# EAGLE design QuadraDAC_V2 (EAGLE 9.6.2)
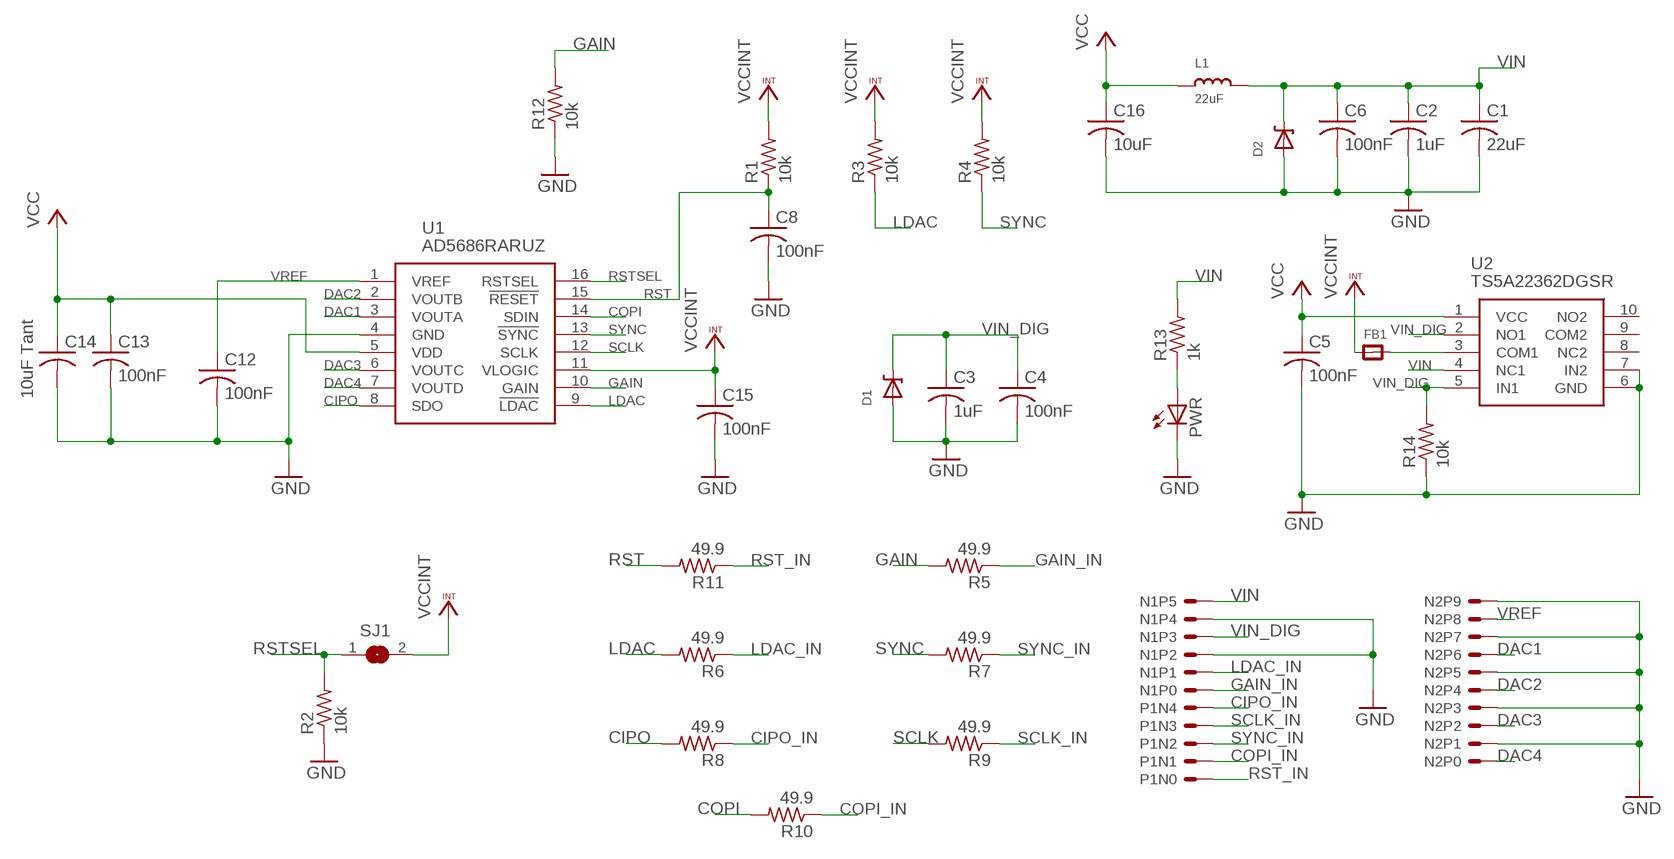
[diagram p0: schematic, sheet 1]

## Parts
C1  22uF  C-USC0603  [C0603]
C2  1uF  C-USC0603  [C0603]
C3  1uF  C-USC0603  [C0603]
C4  100nF  C-USC0603  [C0603]
C5  100nF  C-USC0603  [C0603]
C6  100nF  C-USC0603  [C0603]
C8  100nF  C-USC0603  [C0603]
C12  100nF  C-USC0603  [C0603]
C13  100nF  C-USC0603  [C0603]
C14  10uF Tant  C-USC0805  [C0805]
C15  100nF  C-USC0603  [C0603]
C16  10uF  C-USC0603  [C0603]
D1  DDZ5V6ASF  [DDZ5V6ASF]
D2  DDZ5V6ASF  [DDZ5V6ASF]
FB1  FERRITE_0603  [_0603]
L1  22uF  INDUCTOR0805  [0805]
N1  6PINHEADER  [6PINHEADER]
N2  10PINHEADER  [10PINHEADER]
P1  5PINHEADER  [5PINHEADER]
PWR  LEDCHIPLED_0603  [CHIPLED_0603]
R1  10k  R-US_R0603  [R0603]
R2  10k  R-US_R0603  [R0603]
R3  10k  R-US_R0603  [R0603]
R4  10k  R-US_R0603  [R0603]
R5  49.9  R-US_R0603  [R0603]
R6  49.9  R-US_R0603  [R0603]
R7  49.9  R-US_R0603  [R0603]
R8  49.9  R-US_R0603  [R0603]
R9  49.9  R-US_R0603  [R0603]
R10  49.9  R-US_R0603  [R0603]
R11  49.9  R-US_R0603  [R0603]
R12  10k  R-US_R0603  [R0603]
R13  1k  R-US_R0603  [R0603]
R14  10k  R-US_R0603  [R0603]
SJ1  SOLDERJUMPER  [SOLDERJUMPER_ARROW_NOPASTE]
U1  AD5686RARUZ  [SOP65P640X120-16N]
U2  TS5A22362DGSR  [SOP50P490X110-10N]

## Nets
CIPO: R8.2 U1.8(SDO)
CIPO_IN: P1.N4 R8.1
COPI: R10.2 U1.14(SDIN)
COPI_IN: P1.N1 R10.1
DAC1: N2.P6 U1.3(VOUTA)
DAC2: N2.P4 U1.2(VOUTB)
DAC3: N2.P2 U1.6(VOUTC)
DAC4: N2.P0 U1.7(VOUTD)
GAIN: R5.2 R12.2 U1.10(GAIN)
GAIN_IN: N1.P0 R5.1
GND: C1.2 C2.2 C3.2 C4.2 C5.2 C6.2 C8.2 C12.2 C13.2 C14.2 C15.2 C16.2 D1.P$1(A) D2.P$1(A) N1.P2 N1.P4 N2.P1 N2.P3 N2.P5 N2.P7 N2.P9 PWR.C R2.1 R12.1 R14.1 U1.4(GND) U2.6(GND) U2.7(IN2)
LDAC: R3.1 R6.2 U1.9(!LDAC)
LDAC_IN: N1.P1 R6.1
N$1: PWR.A R13.1
N$4: FB1.2 U2.3(COM1)
RST: C8.1 R1.1 R11.2 U1.15(!RESET)
RST_IN: P1.N0 R11.1
RSTSEL: R2.2 SJ1.1 U1.16(RSTSEL)
SCLK: R9.2 U1.12(SCLK)
SCLK_IN: P1.N3 R9.1
SYNC: R4.1 R7.2 U1.13(!SYNC)
SYNC_IN: P1.N2 R7.1
VCC: C5.1 C13.1 C14.1 C16.1 L1.1 U1.5(VDD) U2.1(VCC)
VCCINT: C15.1 FB1.1 R1.2 R3.2 R4.2 SJ1.2 U1.11(VLOGIC)
VIN: C1.1 C2.1 C6.1 D2.P$2(C) L1.2 N1.P5 R13.2 U2.4(NC1)
VIN_DIG: C3.1 C4.1 D1.P$2(C) N1.P3 R14.2 U2.2(NO1) U2.5(IN1)
VREF: C12.1 N2.P8 U1.1(VREF)
Unconnected: U2.8(NC2) U2.9(COM2) U2.10(NO2)

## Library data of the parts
C1-C6 C8 C12-C16 = rcl:C-US: CAPACITOR, American symbol; SPICEPREFIX: C
D1 D2 = ForceTronics:DDZ5V6ASF: DDZ5V6ASF 5.42 Zener Diode
FB1 = microbuilder:FERRITE: Ferrite Bead
L1 = microbuilder:INDUCTOR: Inductors
N1 = ForceTronics-ForceTronics:6PINHEADER
N2 = ForceTronics-ForceTronics:10PINHEADER
P1 = ForceTronics-ForceTronics:5PINHEADER
PWR = adafruit:LED: LED
R1-R14 = rcl:R-US_: RESISTOR, American symbol; SPICEPREFIX: R
SJ1 = microbuilder:SOLDERJUMPER: SMD Solder JUMPER; BOM: EXCLUDE
U1 = SamacSys_Parts:AD5686RARUZ: AD5686RARUZ, 16 bit DAC Quad SPI, 16-pin TSSOP Source: Datasheet; DESCRIPTION: AD5686RARUZ, 16 bit DAC Quad SPI, 16-pin TSSOP; HEIGHT: 1.2mm; MANUFACTURER_NAME: Analog Devices; MANUFACTURER_PART_NUMBER: AD5686RARUZ; MOUSER_PART_NUMBER: 584-AD5686RARUZ; MOUSER_PRICE-STOCK: https://www.mouser.co.uk/ProductDetail/Analog-Devices/AD5686RARUZ?qs=NmRFExCfTkGcAlYhNpYDVg%3D%3D
U2 = SamacSys_Parts:TS5A22362DGSR: Texas Instruments TS5A22362DGSR, Analogue Switch Dual SPDT, 2.3 5.5 V, 10-Pin VSSOP Source: Datasheet; DESCRIPTION: Texas Instruments TS5A22362DGSR, Analogue Switch Dual SPDT, 2.3 5.5 V, 10-Pin VSSOP; HEIGHT: 1.1mm; MANUFACTURER_NAME: Texas Instruments; MANUFACTURER_PART_NUMBER: TS5A22362DGSR; MOUSER_PART_NUMBER: 595-TS5A22362DGSR; MOUSER_PRICE-STOCK: https://www.mouser.co.uk/ProductDetail/Texas-Instruments/TS5A22362DGSR?qs=snW7ThfrdqwrWVQhLBj0GQ%3D%3D

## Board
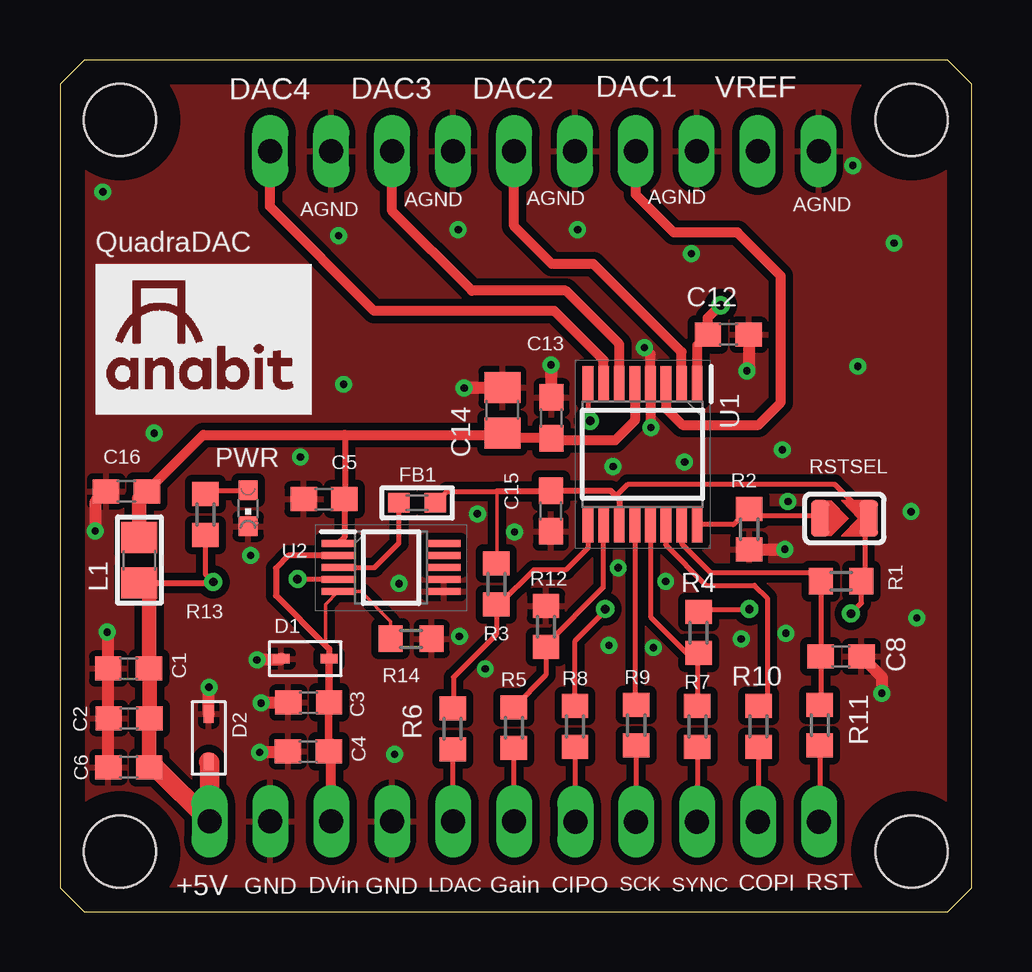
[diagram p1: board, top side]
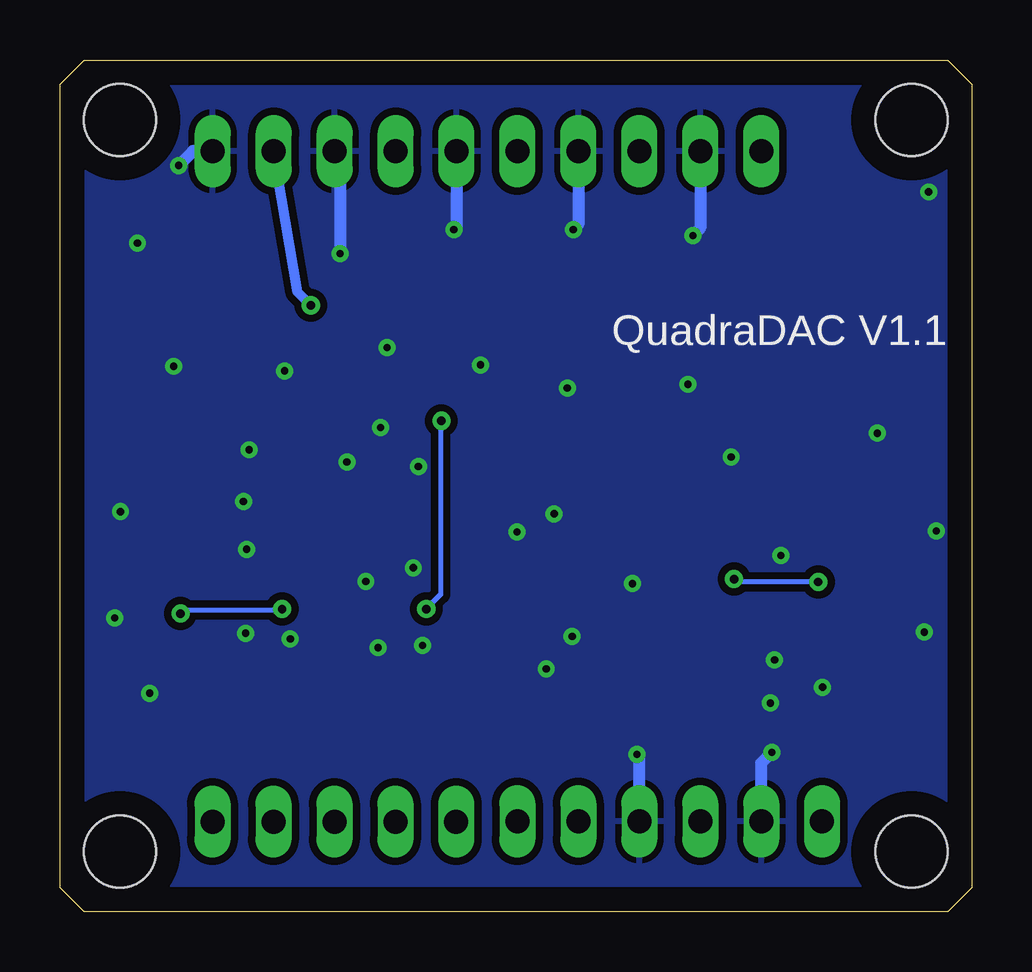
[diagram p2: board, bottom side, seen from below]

Size 38 x 35.5 mm. Coordinates in mm from the lower left corner, seen from the top.
Outline: 38,1 38,34.5 37,35.5 1,35.5 0,34.5 0,1 1,0 37,0 38,1
Copper layers (1*16): Top 0.035mm / dielectric 1.5mm / Bottom 0.035mm
Design rules "default *": minimum track width 6mil, minimum drill 0.3mm, track to track 6mil, track to pad 6mil, pad to pad 6mil, via to via 6mil, smd to smd 6mil, copper to edge 40mil, drill to drill 6mil, minimum pad ring 10mil, minimum via ring 8mil, stop-mask expansion 4mil, vias tented up to drill 0mil, thermal gap 10mil
Holes 3 mm at 2.5,2.5 35.5,2.5 2.5,33 35.5,33

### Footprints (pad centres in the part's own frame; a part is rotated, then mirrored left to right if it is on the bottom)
C0603 = smd 1.1 x 1: 1 -0.85,0; 2 0.85,0
C0805 = smd 1.3 x 1.5: 1 -0.95,0; 2 0.95,0
DDZ5V6ASF = smd 0.71 x 0.41: P$1 0,0; P$2 1.99,0
_0603 = smd 0.9 x 0.8: 1 -0.762,0; 2 0.762,0
0805 = smd 1.3 x 1.5: 1 -0.95,0; 2 0.95,0
6PINHEADER = drill 1 long: P0 1.27,-1.778; P1 3.81,-1.778; P2 6.35,-1.778; P3 8.89,-1.778; P4 11.43,-1.778; P5 13.97,-1.778
10PINHEADER = drill 1 long: P0 1.27,-3.81; P1 3.81,-3.81; P2 6.35,-3.81; P3 8.89,-3.81; P4 11.43,-3.81; P5 13.97,-3.81; P6 16.51,-3.81; P7 19.05,-3.81; P8 21.59,-3.81; P9 24.13,-3.81
5PINHEADER = drill 1 long: N0 -5.08,0; N1 -2.54,0; N2 0,0; N3 2.54,0; N4 5.08,0
CHIPLED_0603 = smd 0.8 x 0.8: A 0,-0.75; C 0,0.75
R0603 = smd 1 x 1.1: 1 -0.85,0; 2 0.85,0
SOLDERJUMPER_ARROW_NOPASTE = smd 0.762 x 1.524: 1 -1.016,0; 2 1.016,0
SOP65P640X120-16N = smd 1.475 x 0.45: 1 -2.938,2.275; 2 -2.938,1.625; 3 -2.938,0.975; 4 -2.938,0.325; 5 -2.938,-0.325; 6 -2.938,-0.975; 7 -2.938,-1.625; 8 -2.938,-2.275; 9 2.938,-2.275; 10 2.938,-1.625; 11 2.938,-0.975; 12 2.938,-0.325; 13 2.938,0.325; 14 2.938,0.975; 15 2.938,1.625; 16 2.938,2.275
SOP50P490X110-10N = smd 1.4 x 0.3: 1 -2.2,1; 2 -2.2,0.5; 3 -2.2,0; 4 -2.2,-0.5; 5 -2.2,-1; 6 2.2,-1; 7 2.2,-0.5; 8 2.2,0; 9 2.2,0.5; 10 2.2,1

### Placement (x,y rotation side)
C1  2.86,10.13 180 top
C2  2.88,8.06 180 top
C3  10.37,8.71 180 top
C4  10.35,6.68 180 top
C5  11.01,17.19 180 top
C6  2.87,6.02 180 top
C8  32.56,10.63 0 top
C12  27.86,24.05 0 top
C13  20.49,20.58 90 top
C14  18.44,20.9 90 top
C15  20.46,16.7 270 top
C16  2.77,17.52 180 top
D1  9.22,10.54 0 top
D2  6.2,8.23 270 top
FB1  14.89,17.04 180 top
L1  3.31,14.65 270 top
N1  20.2,1.98 180 top
N2  7.5,35.51 0 top
P1  26.56,3.75 180 top
PWR  7.84,16.81 180 top
R1  32.56,13.77 0 top
R2  28.73,15.94 90 top
R3  18.19,13.66 90 top
R4  26.62,11.63 90 top
R5  18.92,7.67 90 top
R6  16.37,7.62 90 top
R7  26.57,7.72 90 top
R8  21.47,7.72 90 top
R9  24.02,7.77 90 top
R10  29.12,7.72 90 top
R11  31.67,7.77 90 top
R12  20.26,11.88 270 top
R13  6.07,16.55 270 top
R14  14.64,11.37 180 top
SJ1  32.7,16.39 0 top
U1  24.29,19.06 270 top
U2  13.8,14.34 0 top

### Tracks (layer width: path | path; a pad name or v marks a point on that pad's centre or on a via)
CIPO  (via drill 0.35)
  Top 0.2: U1.8 22.02,20.46 v22.1,20.46 | v22.73,12.61 22.53,12.41 22.53,12.35 21.47,11.29 R8.2
  Bottom 0.2: v22.73,12.61 22.13,13.21 22.13,20.35 22.1,20.38 v22.1,20.46
CIPO_IN
  Top 0.2: P1.N4 R8.1
COPI
  Top 0.2: U1.14 25.25,16.11 25.25,15.28 26.93,13.6 28.95,13.6 29.48,13.07 29.48,8.93 R10.2
COPI_IN
  Top 0.2: R10.1 29.12,3.88 P1.N1
DAC1
  Top 0.406: U1.3 25.27,20.98 25.95,20.29 29.12,20.29 30.05,21.22 30.05,26.5 28.24,28.31 25.59,28.31 24.01,29.89 N2.P6
DAC2
  Top 0.2: U1.2 25.9,22.01
  Top 0.406: U1.2 25.91,23.32 22.24,27 20.51,27 18.93,28.58 N2.P4
DAC3
  Top 0.406: U1.6 23.32,23.66 21.09,25.88 17.17,25.88 13.85,29.2 N2.P2
DAC4
  Top 0.406: U1.7 22.66,22.98 20.61,25.04 13.1,25.04 8.75,29.39 8.75,31.68 N2.P0
GAIN
  Top 0.2: U1.10 22.64,16.1 22.64,13.51 20.26,11.12 R12.2 20.26,9.86 R5.2
GAIN_IN
  Top 0.2: N1.P0 R5.1
GND  (via drill 0.3)
  Top 0.305: 24.61,20.2 v24.63,20.18
  Top 0.406: 24.61,20.2 U1.4 24.61,23.25 v24.36,23.51
  Top 0.508: C6.2 C2.2 2.01,8.08 C1.2 2.01,11.61 v1.97,11.65 | C16.2 1.47,17.07 v1.47,15.87 | D2.P$1 v6.2,9.34 v6.21,9.35 | C3.2 9.5,8.69 v8.39,8.69 | D1.P$1 9.17,10.49 v8.21,10.49 | C4.2 9.46,6.64 v8.32,6.64 | C8.2 34.26,9.78 v34.26,9.1 | R2.1 v30.21,15.09 v30.22,15.1 | C12.2 28.71,22.62 v28.63,22.54 | C14.2 18.41,21.82 v16.85,21.82 | C13.2 20.49,22.77 v20.47,22.79
  Bottom 0.508: N1.P2 13.85,6.45 v13.95,6.55 | N1.P4 8.77,6.19 v8.32,6.64 | v33.05,31.1 32.45,31.7 N2.P9 | N2.P1 11.31,28.49 v11.62,28.18 | v16.6,28.43 16.39,28.64 N2.P3 | N2.P5 21.47,28.54 v21.58,28.43 | N2.P7 26.32,31.47 v26.32,27.43
  other vias: 18.95,15.82 22.88,11.09 17.73,10.12 23.06,18.55 1.79,30 11.82,21.98 33.26,22.73 3.93,19.94 34.77,27.86 35.72,12.24 30.35,17.09 16.65,11.47 23.27,14.33 7.95,14.84 10.02,18.95 14.13,13.67 17.4,16.58 26.04,18.74 30.12,19.25 24.74,11 25.25,13.76 28.4,11.36 30.26,11.6 35.48,16.67
  pour Bottom (isolate 0.305): -0.75,-0.5 -0.75,37.75 38.75,37.75 38.75,0.25 37.75,-0.75 -0.5,-0.75
  pour Top (isolate 0.305): -1.75,37.25 38.75,37.25 39,37 39,0 38.25,-0.75 -1,-0.75 -1.75,0
LDAC
  Top 0.2: U1.9 22.02,15.16 21.1,14.25 19.75,14.25 18.31,12.81 R3.1 18.19,11.56 16.4,9.77 16.4,8.5 R6.2
LDAC_IN
  Top 0.2: R6.1 16.39,6.75 N1.P1
N$1
  Top 0.203: R13.1 6.23,17.56 PWR.A
N$4
  Top 0.203: U2.3 13.11,14.34 14.13,15.36 FB1.2
RST
  Top 0.2: U1.15 25.91,15.35 27.14,14.12 31.36,14.12 R1.1 C8.1 31.71,8.66 R11.2
RST_IN
  Top 0.2: R11.1 31.67,3.89 P1.N0
RSTSEL
  Top 0.2: U1.16 26.57,16.13 28.07,16.13 R2.2 29.04,16.48 | SJ1.1 31.59,16.48 29.04,16.48 | 29.04,16.48 28.75,16.48
SCLK
  Top 0.2: U1.12 23.96,8.68 R9.2
SCLK_IN
  Top 0.2: R9.1 P1.N3
SYNC
  Top 0.2: U1.13 24.61,12.29 26.12,10.78 R4.1 26.57,10.73 R7.2
SYNC_IN
  Top 0.2: R7.1 26.57,3.87 P1.N2
VCC
  Top 0.254: 18.66,19.73 18.52,19.88 C14.1 18.21,19.72 | 11.88,19.88 11.88,17.21 C5.1 11.86,15.6 U2.1
  Top 0.406: U1.5 23.96,20.46 23.14,19.64 20.58,19.64 C13.1 18.66,19.73 | C16.1 5.97,19.88 11.88,19.88 18.52,19.88
  Top 0.61: L1.1 3.31,17.21 C16.1
VCCINT  (via drill 0.35)
  Top 0.152: R3.2 18.22,14.54 18.22,17.52
  Top 0.2: 23.18,17.32 23.68,17.82 32.29,17.82 SJ1.2 33.56,16.23 33.56,13.62 R1.2 33.41,12.86 v32.98,12.43 | R4.2 26.73,12.59 28.72,12.59 v28.74,12.61
  Top 0.203: FB1.1 16.13,17.52 18.22,17.52
  Top 0.254: 18.22,17.52 20.43,17.52 C15.1 22.95,17.55 23.18,17.32 23.32,17.18 U1.11
  Bottom 0.2: v28.74,12.61 28.78,12.57 32.83,12.57 v32.98,12.43
VIN  (via drill 0.35)
  Top 0.203: v9.9,13.86 11.58,13.86 U2.4 | v6.39,13.74 6.07,14.06 R13.2
  Top 0.254: L1.2 6.26,13.7 6.3,13.74 v6.39,13.74
  Top 0.508: 6.23,6.24 D2.P$2
  Top 0.61: 3.97,6.02 C6.1 C2.1 3.73,10.11 C1.1 | C1.1 3.97,9.97 | C1.1 3.71,13.3 L1.2
  Top 0.813: D2.P$2 6.23,6.21 N1.P5 3.97,6.02
  Bottom 0.203: v6.39,13.74 9.78,13.74 v9.9,13.86
VIN_DIG
  Top 0.152: 11.07,11.1 11.07,12.81 U2.5 12.55,13.34 13.79,12.1 R14.2
  Top 0.254: U2.2 9.53,14.84 9,14.31 9,13.17 11.07,11.1 11.22,10.95 D1.P$2
  Top 0.305: C4.1 11.2,8.69 C3.1 D1.P$2
  Top 0.406: N1.P3 11.31,6.57 | 11.31,6.57 11.31,7.02 | C4.1 11.31,6.57
VREF  (via drill 0.35)
  Top 0.2: 26.62,23.98 26.94,23.98 C12.1 27.05,24.05 27.05,24.06
  Top 0.305: U1.1 26.62,22.05
  Top 0.406: U1.1 26.57,23.61 26.94,23.98 | C12.1 27.01,24.76 27.52,25.27 v27.54,25.27
  Bottom 0.406: v27.54,25.27 28.09,25.82 N2.P8

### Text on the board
tNames: DAC4 | DAC3 | DAC2 | DAC1 | VREF | AGND | AGND | AGND | AGND | AGND | QuadraDAC | RSTSEL | +5V | GND | DVin | GND | LDAC | Gain | CIPO | SCK | SYNC | COPI | RST
bNames: QuadraDAC V1.1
